FUNCTION "COM_GENER" : VOID
TITLE =
AUTHOR : LD
FAMILY : DESTACK
NAME : GENER
VERSION : 0.1

BEGIN
NETWORK
TITLE =Emergenze ripristinate
//OK
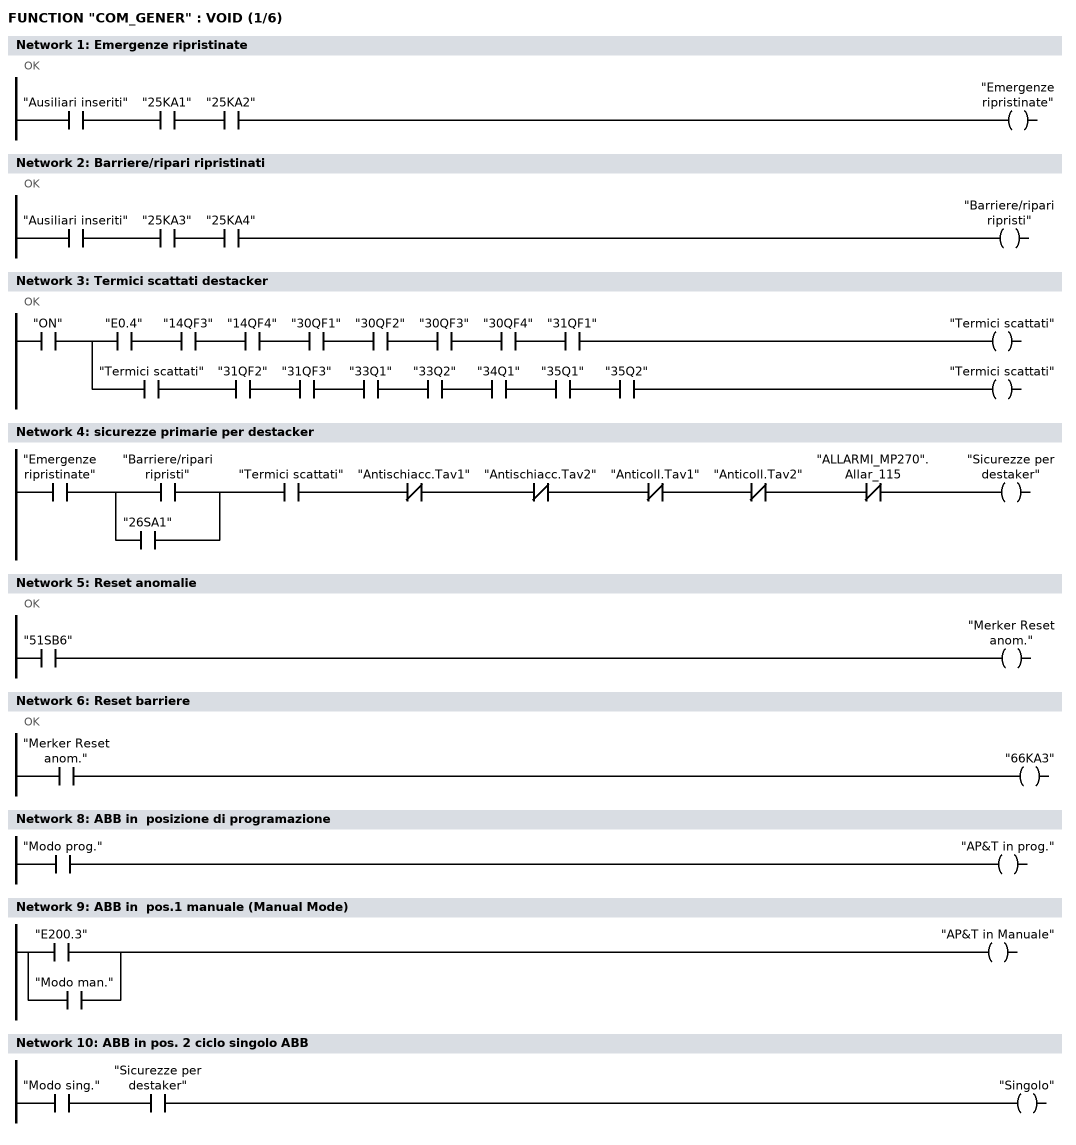
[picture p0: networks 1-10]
      U     "Ausiliari inseriti";
      U     "25KA1";
      U     "25KA2";
      =     "Emergenze ripristinate";
NETWORK
TITLE =Barriere/ripari ripristinati
//OK
      U     "Ausiliari inseriti";
      U     "25KA3";
      U     "25KA4";
      =     "Barriere/ripari ripristi";
NETWORK
TITLE =Termici scattati destacker
//OK
      U     "ON";
      =     L      0.0;
      U     L      0.0;
      U     "E0.4";
      U     "14QF3";
      U     "14QF4";
      U     "30QF1";
      U     "30QF2";
      U     "30QF3";
      U     "30QF4";
      U     "31QF1";
      =     "Termici scattati";
      U     L      0.0;
      U     "Termici scattati";
      U     "31QF2";
      U     "31QF3";
      U     "33Q1";
      U     "33Q2";
      U     "34Q1";
      U     "35Q1";
      U     "35Q2";
      =     "Termici scattati";
NETWORK
TITLE =sicurezze primarie per destacker

      U     "Emergenze ripristinate";
      U(    ;
      O     "Barriere/ripari ripristi";
      O     "26SA1";
      )     ;
      U     "Termici scattati";
      UN    "Antischiacc.Tav1";
      UN    "Antischiacc.Tav2";
      UN    "Anticoll.Tav1";
      UN    "Anticoll.Tav2";
      UN    "ALLARMI_MP270".Allar_115;
      =     "Sicurezze per destaker";
NETWORK
TITLE =Reset anomalie
//OK
      U     "51SB6";
      =     "Merker Reset anom.";
NETWORK
TITLE =Reset barriere
//OK
      U     "Merker Reset anom.";
      =     "66KA3";
NETWORK
TITLE =



NETWORK
TITLE =ABB in  posizione di programazione

      U     "Modo prog.";
      =     "AP&T in prog.";
NETWORK
TITLE =ABB in  pos.1 manuale (Manual Mode)

      O     "E200.3";
      O     "Modo man.";
      =     "AP&T in Manuale";
NETWORK
TITLE =ABB in pos. 2 ciclo singolo ABB

      U     "Modo sing.";
      U     "Sicurezze per destaker";
      =     "Singolo";
NETWORK
TITLE =ABB in pos. 4 auto (Automatic Mode)
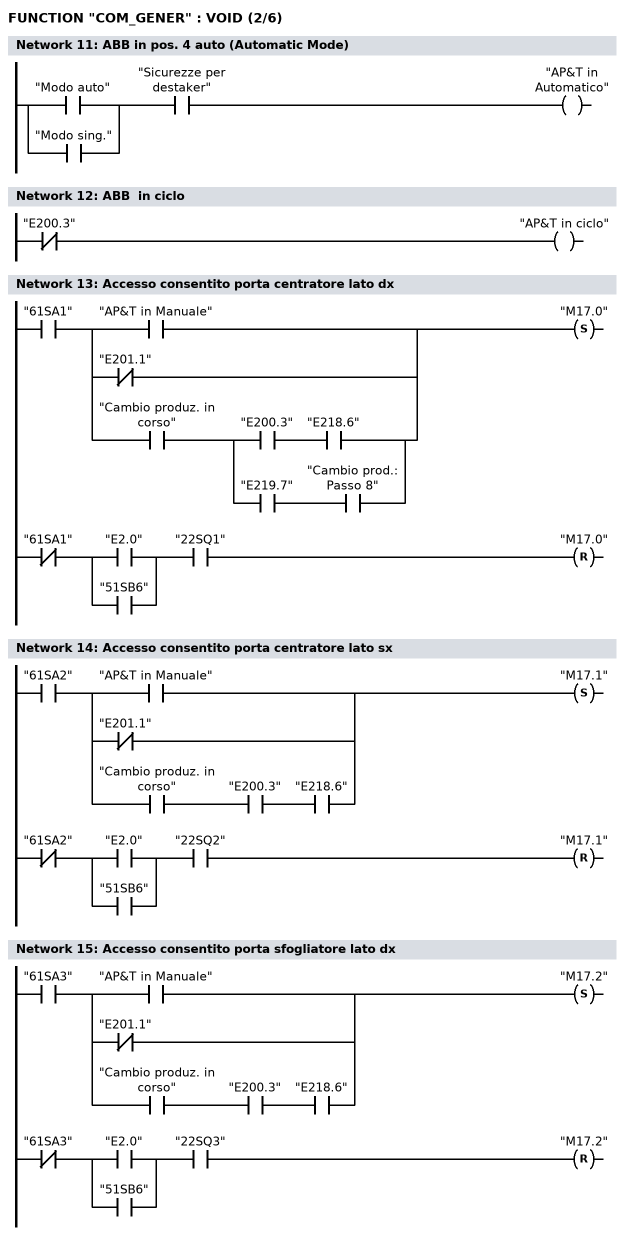
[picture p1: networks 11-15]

      U(    ;
      O     "Modo auto";
      O     "Modo sing.";
      )     ;
      U     "Sicurezze per destaker";
      =     "AP&T in Automatico";
NETWORK
TITLE =ABB  in ciclo

      UN    "E200.3";
      =     "AP&T  in ciclo";
NETWORK
TITLE =Accesso consentito porta centratore lato dx

      U     "61SA1";
      U(    ;
      O     "AP&T in Manuale";
      ON    "E201.1";
      O     ;
      U     "Cambio produz. in corso";
      U(    ;
      U     "E200.3";
      U     "E218.6";
      O     ;
      U     "E219.7";
      U     "Cambio prod.: Passo 8";
      )     ;
      )     ;
      S     "M17.0";
      UN    "61SA1";
      U(    ;
      O     "E2.0";
      O     "51SB6";
      )     ;
      U     "22SQ1";
      R     "M17.0";
      NOP   0;
NETWORK
TITLE =Accesso consentito porta centratore lato sx

      U     "61SA2";
      U(    ;
      O     "AP&T in Manuale";
      ON    "E201.1";
      O     ;
      U     "Cambio produz. in corso";

      U     "E200.3";
      U     "E218.6";
      )     ;
      S     "M17.1";
      UN    "61SA2";
      U(    ;
      O     "E2.0";
      O     "51SB6";
      )     ;
      U     "22SQ2";
      R     "M17.1";
      NOP   0;
NETWORK
TITLE =Accesso consentito porta sfogliatore lato dx

      U     "61SA3";
      U(    ;
      O     "AP&T in Manuale";
      ON    "E201.1";
      O     ;
      U     "Cambio produz. in corso";
      U     "E200.3";
      U     "E218.6";
      )     ;
      S     "M17.2";
      UN    "61SA3";
      U(    ;
      O     "E2.0";
      O     "51SB6";
      )     ;
      U     "22SQ3";
      R     "M17.2";
      NOP   0;
NETWORK
TITLE =Accesso consentito porta sfogliatore lato sx
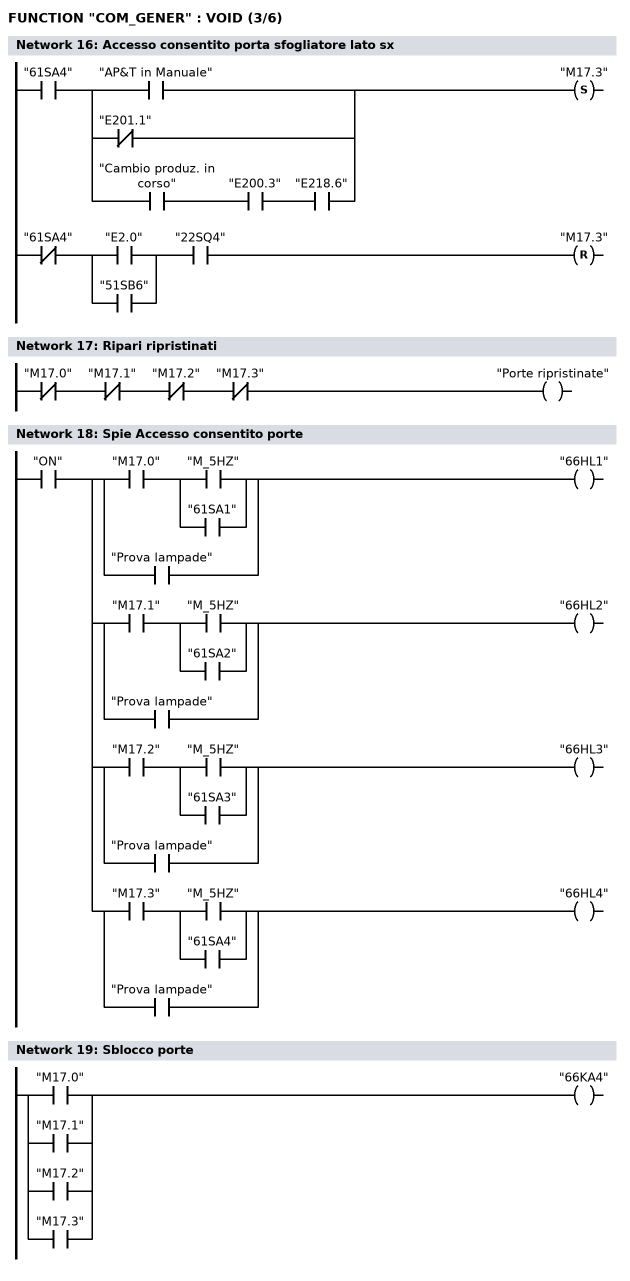
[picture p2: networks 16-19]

      U     "61SA4";
      U(    ;
      O     "AP&T in Manuale";
      ON    "E201.1";
      O     ;
      U     "Cambio produz. in corso";
      U     "E200.3";
      U     "E218.6";
      )     ;
      S     "M17.3";
      UN    "61SA4";
      U(    ;
      O     "E2.0";
      O     "51SB6";
      )     ;
      U     "22SQ4";
      R     "M17.3";
      NOP   0;
NETWORK
TITLE =Ripari ripristinati

      UN    "M17.0";
      UN    "M17.1";
      UN    "M17.2";
      UN    "M17.3";
      =     "Porte ripristinate";
NETWORK
TITLE =Spie Accesso consentito porte

      U     "ON";
      =     L      0.0;
      U     L      0.0;
      U(    ;
      U     "M17.0";
      U(    ;
      O     "M_5HZ";
      O     "61SA1";
      )     ;
      O     "Prova lampade";
      )     ;
      =     "66HL1";
      U     L      0.0;
      U(    ;
      U     "M17.1";
      U(    ;
      O     "M_5HZ";
      O     "61SA2";
      )     ;
      O     "Prova lampade";
      )     ;
      =     "66HL2";
      U     L      0.0;
      U(    ;
      U     "M17.2";
      U(    ;
      O     "M_5HZ";
      O     "61SA3";
      )     ;
      O     "Prova lampade";
      )     ;
      =     "66HL3";
      U     L      0.0;
      U(    ;
      U     "M17.3";
      U(    ;
      O     "M_5HZ";
      O     "61SA4";
      )     ;
      O     "Prova lampade";
      )     ;
      =     "66HL4";
NETWORK
TITLE =Sblocco porte

      O     "M17.0";
      O     "M17.1";
      O     "M17.2";
      O     "M17.3";
      =     "66KA4";
NETWORK
TITLE =Tavola 1 : Sicurezza cancelletto
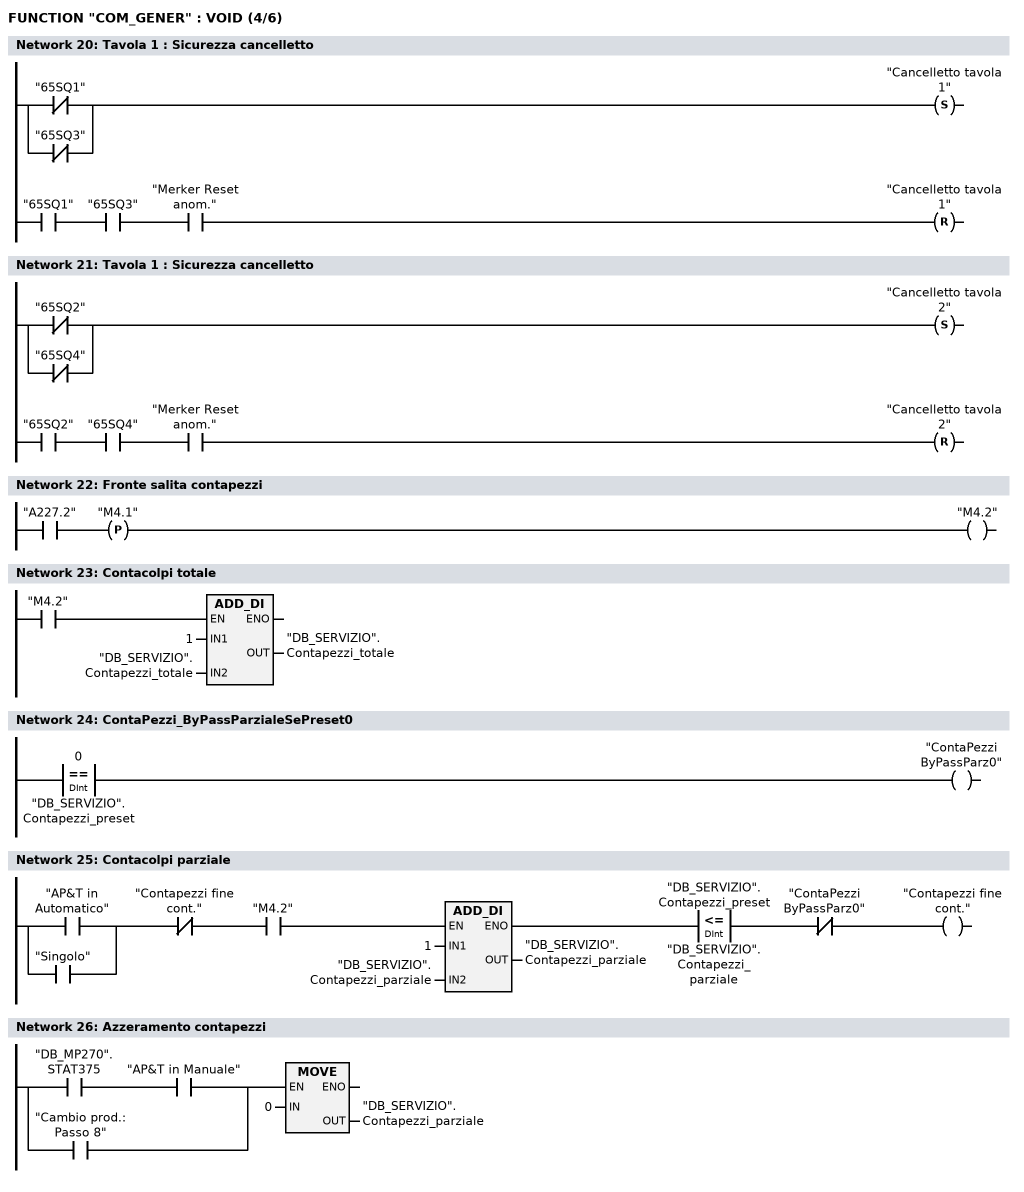
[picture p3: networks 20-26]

      U(    ;
      ON    "65SQ1";
      ON    "65SQ3";


      )     ;
      S     "Cancelletto tavola 1";
      U     "65SQ1";
      U     "65SQ3";
      U     "Merker Reset anom.";
      R     "Cancelletto tavola 1";
      NOP   0;
NETWORK
TITLE =Tavola 1 : Sicurezza cancelletto



      U(    ;
      ON    "65SQ2";
      ON    "65SQ4";
      )     ;
      S     "Cancelletto tavola 2";
      U     "65SQ2";
      U     "65SQ4";
      U     "Merker Reset anom.";
      R     "Cancelletto tavola 2";
      NOP   0;
NETWORK
TITLE =Fronte salita contapezzi

      U     "A227.2";
      FP    "M4.1";
      =     "M4.2";
NETWORK
TITLE =Contacolpi totale

      U     "M4.2";
      SPBNB _001;

      L     1;
      L     "DB_SERVIZIO".Contapezzi_totale;
      +D    ;
      T     "DB_SERVIZIO".Contapezzi_totale;
_001: NOP   0;

NETWORK
TITLE =ContaPezzi_ByPassParzialeSePreset0


      L     0;
      L     "DB_SERVIZIO".Contapezzi_preset;
      ==D   ;
      =     "ContaPezzi ByPassParz0";




NETWORK
TITLE =Contacolpi parziale


      U(    ;
      O     "AP&T in Automatico";
      O     "Singolo";
      )     ;
      UN    "Contapezzi fine cont.";
      U     "M4.2";
      SPBNB M006;
      L     1;
      L     "DB_SERVIZIO".Contapezzi_parziale;
      +D    ;
      T     "DB_SERVIZIO".Contapezzi_parziale;
      UN    OV;
      SAVE  ;
      CLR   ;
M006: U     BIE;
      U(    ;
      L     "DB_SERVIZIO".Contapezzi_preset;
      L     "DB_SERVIZIO".Contapezzi_parziale;
      <=D   ;
      )     ;
      UN    "ContaPezzi ByPassParz0";
      =     "Contapezzi fine cont.";



NETWORK
TITLE =Azzeramento contapezzi

      U(    ;
      U     "DB_MP270".STAT375;
      U     "AP&T in Manuale";
      O     "Cambio prod.: Passo 8";
      )     ;
      SPBNB _002;
      L     0;
      T     "DB_SERVIZIO".Contapezzi_parziale;
_002: NOP   0;
NETWORK
TITLE =ciclo in corso visualizza su MP270
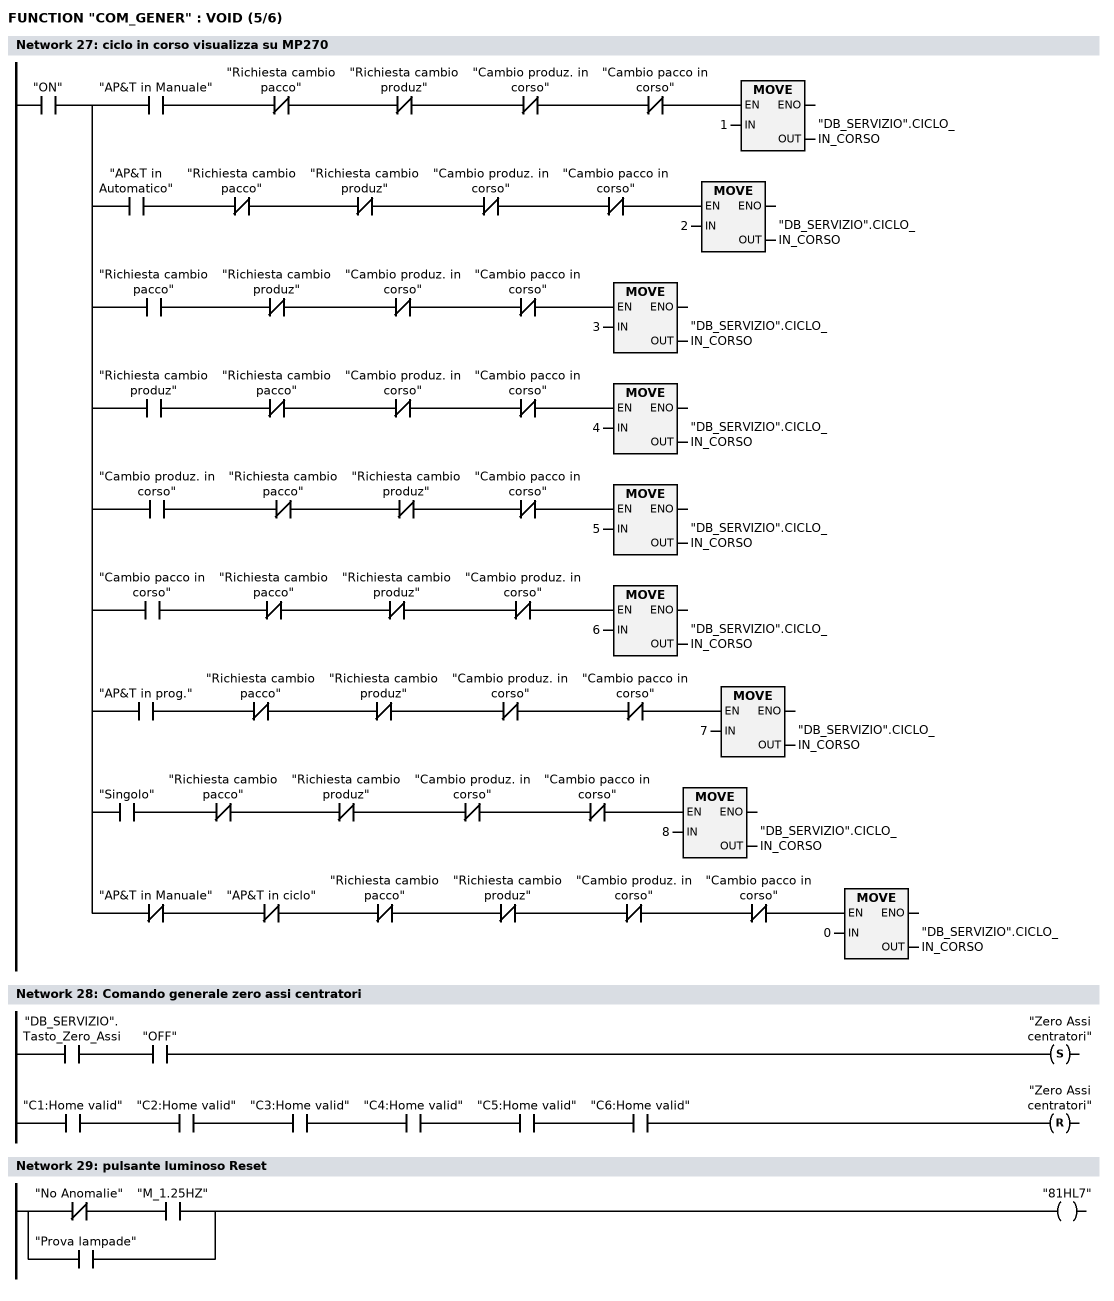
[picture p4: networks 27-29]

      U     "ON";
      =     L      0.0;
      U     L      0.0;
      U     "AP&T in Manuale";
      UN    "Richiesta cambio pacco";
      UN    "Richiesta cambio produz";
      UN    "Cambio produz. in corso";
      UN    "Cambio pacco in corso";
      SPBNB _003;
      L     1;
      T     "DB_SERVIZIO".CICLO_IN_CORSO;
_003: NOP   0;
      U     L      0.0;
      U     "AP&T in Automatico";
      UN    "Richiesta cambio pacco";
      UN    "Richiesta cambio produz";
      UN    "Cambio produz. in corso";
      UN    "Cambio pacco in corso";
      SPBNB _004;
      L     2;
      T     "DB_SERVIZIO".CICLO_IN_CORSO;
_004: NOP   0;
      U     L      0.0;
      U     "Richiesta cambio pacco";
      UN    "Richiesta cambio produz";
      UN    "Cambio produz. in corso";
      UN    "Cambio pacco in corso";
      SPBNB _005;
      L     3;
      T     "DB_SERVIZIO".CICLO_IN_CORSO;
_005: NOP   0;
      U     L      0.0;
      U     "Richiesta cambio produz";
      UN    "Richiesta cambio pacco";
      UN    "Cambio produz. in corso";
      UN    "Cambio pacco in corso";
      SPBNB _006;
      L     4;
      T     "DB_SERVIZIO".CICLO_IN_CORSO;
_006: NOP   0;
      U     L      0.0;
      U     "Cambio produz. in corso";
      UN    "Richiesta cambio pacco";
      UN    "Richiesta cambio produz";
      UN    "Cambio pacco in corso";
      SPBNB _007;
      L     5;
      T     "DB_SERVIZIO".CICLO_IN_CORSO;
_007: NOP   0;
      U     L      0.0;
      U     "Cambio pacco in corso";
      UN    "Richiesta cambio pacco";
      UN    "Richiesta cambio produz";
      UN    "Cambio produz. in corso";
      SPBNB _008;
      L     6;
      T     "DB_SERVIZIO".CICLO_IN_CORSO;
_008: NOP   0;
      U     L      0.0;
      U     "AP&T in prog.";
      UN    "Richiesta cambio pacco";
      UN    "Richiesta cambio produz";
      UN    "Cambio produz. in corso";
      UN    "Cambio pacco in corso";
      SPBNB _009;
      L     7;
      T     "DB_SERVIZIO".CICLO_IN_CORSO;
_009: NOP   0;
      U     L      0.0;
      U     "Singolo";
      UN    "Richiesta cambio pacco";
      UN    "Richiesta cambio produz";
      UN    "Cambio produz. in corso";
      UN    "Cambio pacco in corso";
      SPBNB _00a;
      L     8;
      T     "DB_SERVIZIO".CICLO_IN_CORSO;
_00a: NOP   0;
      U     L      0.0;
      UN    "AP&T in Manuale";
      UN    "AP&T  in ciclo";
      UN    "Richiesta cambio pacco";
      UN    "Richiesta cambio produz";
      UN    "Cambio produz. in corso";
      UN    "Cambio pacco in corso";
      SPBNB _00b;
      L     0;
      T     "DB_SERVIZIO".CICLO_IN_CORSO;
_00b: NOP   0;
NETWORK
TITLE =Comando generale zero assi centratori

      U     "DB_SERVIZIO".Tasto_Zero_Assi;
      U     "OFF";
      S     "Zero Assi centratori";
      U     "C1:Home valid";
      U     "C2:Home valid";
      U     "C3:Home valid";
      U     "C4:Home valid";
      U     "C5:Home valid";
      U     "C6:Home valid";
      R     "Zero Assi centratori";
      NOP   0;
NETWORK
TITLE =pulsante luminoso Reset

      UN    "No Anomalie";
      U     "M_1.25HZ";
      O     "Prova lampade";
      =     "81HL7";
NETWORK
TITLE =pulsante luminoso emergenza da ripristinare
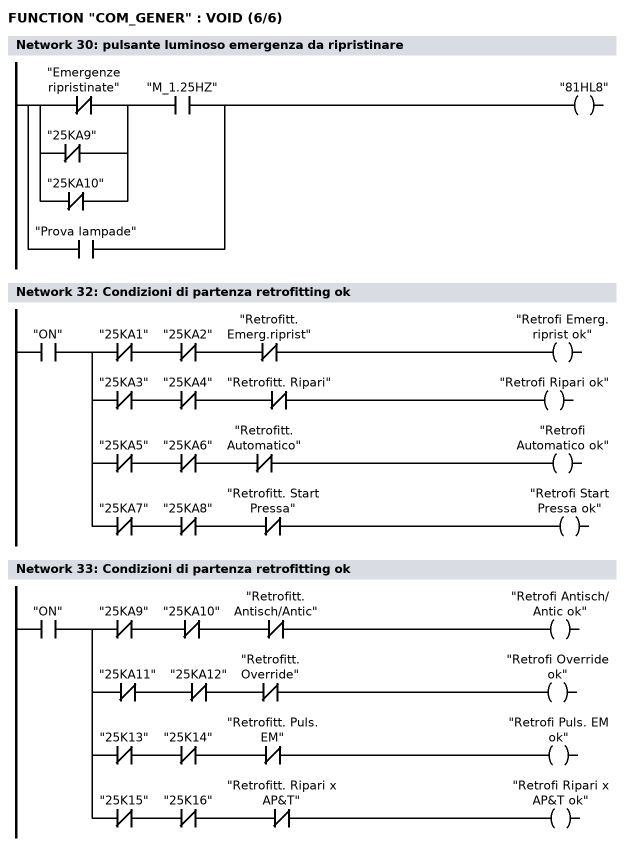
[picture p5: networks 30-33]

      U(    ;
      ON    "Emergenze ripristinate";
      ON    "25KA9";
      ON    "25KA10";
      )     ;
      U     "M_1.25HZ";
      O     "Prova lampade";
      =     "81HL8";
NETWORK
TITLE =



NETWORK
TITLE =Condizioni di partenza retrofitting ok

      U     "ON";
      =     L      0.0;
      U     L      0.0;
      UN    "25KA1";
      UN    "25KA2";
      UN    "Retrofitt. Emerg.riprist";
      =     "Retrofi Emerg.riprist ok";
      U     L      0.0;
      UN    "25KA3";
      UN    "25KA4";
      UN    "Retrofitt. Ripari";
      =     "Retrofi Ripari ok";
      U     L      0.0;
      UN    "25KA5";
      UN    "25KA6";
      UN    "Retrofitt. Automatico";
      =     "Retrofi Automatico ok";
      U     L      0.0;
      UN    "25KA7";
      UN    "25KA8";
      UN    "Retrofitt. Start Pressa";
      =     "Retrofi Start Pressa ok";
NETWORK
TITLE =Condizioni di partenza retrofitting ok

      U     "ON";
      =     L      0.0;
      U     L      0.0;
      UN    "25KA9";
      UN    "25KA10";
      UN    "Retrofitt. Antisch/Antic";
      =     "Retrofi Antisch/Antic ok";
      U     L      0.0;
      UN    "25KA11";
      UN    "25KA12";
      UN    "Retrofitt. Override";
      =     "Retrofi Override ok";
      U     L      0.0;
      UN    "25K13";
      UN    "25K14";
      UN    "Retrofitt. Puls. EM";
      =     "Retrofi Puls. EM ok";
      U     L      0.0;
      UN    "25K15";
      UN    "25K16";
      UN    "Retrofitt. Ripari x AP&T";
      =     "Retrofi Ripari x AP&T ok";
END_FUNCTION

